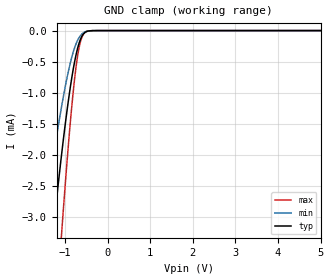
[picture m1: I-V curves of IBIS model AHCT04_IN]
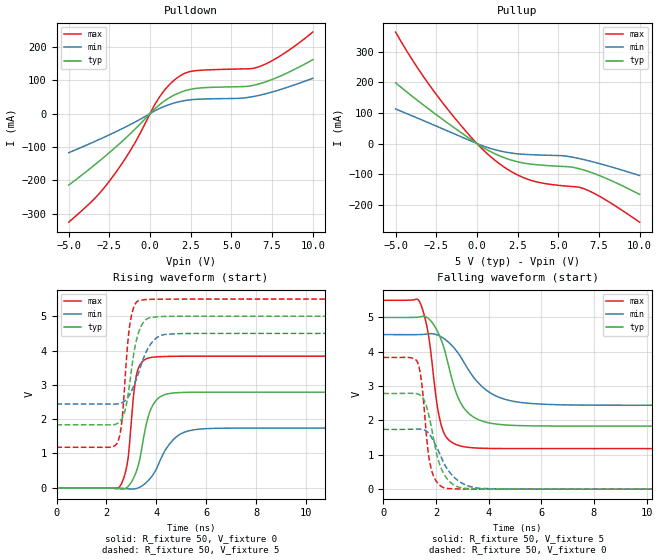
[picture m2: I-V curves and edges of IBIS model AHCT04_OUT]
| TEXAS INSTRUMENTS INCORPORATED
| Standard Linear and Logic Group
| IBIS Model of SN74AHCT1G04
| SINGLE INVERTER GATE
| This file contains package information for the following:
|  SOT 5-pin (DBV) package as [Component] AHCT04_DBV
|  SOT 5-pin (DCK) package as [Component] AHCT04_DCK
| This device can be powered at the following Vccs:
|  5 volt Vcc
| This file provides unique models under the [Model Selector] for each Vcc.
| For operation at a specific Vcc, select the appropriate model after each
| [Model Selector] keyword.
[IBIS Ver]   3.2
[Comment char]  |_char
[File Name]   sn74ahct1g04.ibs
[File Rev]   1.1 | j_die
[Date]   October 25, 2007
[Source]   Data created from TI-SPICE simulations at TI-SLL.
[Notes]   The following is an IBIS list for the SN74AHCT1G04.
   Please contact sllibis@ti.com with questions and
   comments concerning SLL IBIS models.
   - FILE REV HISTORY
   - 1.1 Release IBIS file on 11/9/07
   - Power clamp data deleted as there is no power-clamp diode.
[Disclaimer] Property of Texas Instruments Incorporated.  Unauthorized
   reproduction and/or distribution is strictly prohibited.
   This product is protected under copyright law.
   Created  2007, (C) Copyright  2007, Texas Instruments
   Incorporated, All Rights Reserved
   UNLESS THERE IS A SIGNED, WRITTEN AGREEMENT TO THE
   CONTRARY, TEXAS INSTRUMENTS (TI) IS PROVIDING THE IBIS
   MODELS  AND WITHOUT ANY WARRANTY, EXPRESSED OR
   IMPLIED.  TI assumes no liability for:
   1) the accuracy of the IBIS models provided to your
   company;
   2) the proper functioning of these IBIS Models in your
   design or for any resulting applications; or
   3) infringement of patents, copyrights or intellectual
   property rights resulting from your use of these IBIS
   models.
   TI provides IBIS Models as a service to our customers.
   You and your company shall not distribute, sell or give
   these models to anyone else without prior written
   permission from TI.
   TI reserves the right to make changes to our products or
   to discontinue any semiconductor product or service
   without notice, and advises our customers to obtain the
   latest version of relevant information to verify, before
   placing orders, that the information being relied on is
   current.
   Please be aware that your receipt and use of the IBIS
   information provided shall serve as acceptance of these
   terms and conditions.  If you do not accept these terms,
   you should return or destroy the IBIS models and any
   other accompanying information immediately.
| Component SN74AHCT1G04_DBV 5-PIN SOT
[Component]   SN74AHCT1G04_DBV
[Manufacturer]   Texas Instruments, Inc.
[Package]
|   typ   min   max
R_pkg   2.500e-02   2.100e-02   2.900e-02
L_pkg   1.529e-09   1.312e-09   1.906e-09
C_pkg   1.560e-13   1.100e-13   2.400e-13
[Pin]   signal_name   model_name   R_pin   L_pin   C_pin
1   NC   NC   2.100e-02   1.511e-09   1.440e-13
2   A   AHCT04_IN   2.300e-02   1.312e-09   1.380e-13
3   GND   GND   2.900e-02   1.906e-09   2.400e-13
4   Y   AHCT04_OUT   2.600e-02   1.541e-09   1.500e-13
5   VCC   POWER   2.500e-02   1.374e-09   1.100e-13
| Component SN74AHCT1G04_DCK 5-PIN SOT
[Component]   SN74AHCT1G04_DCK
[Manufacturer]   Texas Instruments, Inc.
[Package]
|   typ   min   max
R_pkg   2.000e-02   1.700e-02   2.500e-02
L_pkg   9.980e-10   8.810e-10   1.069e-09
C_pkg   1.460e-13   1.180e-13   2.050e-13
[Pin]   signal_name   model_name   R_pin   L_pin   C_pin
1   NC   NC   1.900e-02   1.069e-09   1.620e-13
2   A   AHCT04_IN   1.800e-02   8.810e-10   1.210e-13
3   GND   GND   1.700e-02   1.031e-09   2.050e-13
4   Y   AHCT04_OUT   2.000e-02   9.600e-10   1.240e-13
5   VCC   POWER   2.500e-02   1.049e-09   1.180e-13
| Models and submodels in the file (2): AHCT04_IN (Input), AHCT04_OUT (Output)
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[Model]   AHCT04_IN
Model_type  Input
Vinl=0.8
Vinh=2.0
| variable   typ   min   max
C_comp   1.07pF   0.88pF   1.17pF
[Temperature Range]   40   100   -40
| Ambient temperature   25   85   -40
[Voltage range]   5   4.5   5.5
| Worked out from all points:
|   GND clamp passes 1 mA (typ) near -0.89 V on its own axis
[GND Clamp]
| AHCT04_IN
|   Voltage   I(typ)   I(min)   I(max)
-5V       -39.05mA   -25.88mA   -50.64mA
-1.54V    -5.118mA   -3.294mA   -8.041mA
-1.49V    -4.743mA   -3.046mA   -7.491mA
-1.28V    -3.254mA   -2.059mA   -5.253mA
-1.08V    -1.989mA   -1.219mA   -3.261mA
-900mV    -1.024mA   -591uA     -1.667mA
-775mV    -501.2uA   -275.4uA   -773.8uA
-720mV    -326.3uA   -178.4uA   -476uA
-660mV    -181.4uA   -102.3uA   -240.9uA
-610mV    -98.63uA   -59.63uA   -118uA
-540mV    -34.66uA   -23.86uA   -34.5uA
5V        17.64nA    1.142nA    163.4nA
[Model]   AHCT04_OUT
Model_type  Output
Vref =   0
Rref =   1000
Cref =   50p
Vmeas =   1.5
| variable   typ   min   max
C_comp   3.84pF   2.05pF   6.98pF
| C_pullup   3.33pF   2.05pF   4.35pF
| C_pulldown   4.35pF   2.74pF   6.98pF
[Temperature Range]   40   100   -40
| Ambient temperature   25   85   -40
[Voltage range]   5   4.5   5.5
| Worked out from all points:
|   slope of the pulldown table from 0 to 0.75 V, typ, clamps not added: 22.7 ohm
|   slope of the pullup table from 0 to 0.75 V, typ, clamps not added: 31.3 ohm
|   rising waveform, R_fixture 50, V_fixture 0: 20-80 % time 509ps typ, 836ps min, 304ps max; typ from 0 V to 2.79 V
|   falling waveform, R_fixture 50, V_fixture 5: 20-80 % time 783ps typ, 1.25ns min, 462ps max; typ from 5 V to 1.84 V
|   rising waveform, R_fixture 50, V_fixture 5: 20-80 % time 414ps typ, 660ps min, 281ps max; typ from 1.84 V to 5 V
|   falling waveform, R_fixture 50, V_fixture 0: 20-80 % time 522ps typ, 776ps min, 309ps max; typ from 2.79 V to 0 V
[Pulldown]
| AHCT04_OUT
|   Voltage   I(typ)   I(min)   I(max)
-5V       -214.3mA   -117.4mA   -325.8mA
-3.425V   -154.6mA   -84.24mA   -255.7mA
-2.375V   -111.7mA   -60.8mA    -194.5mA
-1.035V   -51.93mA   -28.28mA   -96.41mA
515mV     23.92mA    13.69mA    44.79mA
1.035V    42.89mA    24.61mA    78.63mA
1.59V     58.05mA    33.27mA    104.4mA
2.66V     74.47mA    42.18mA    127.9mA
5.55V     80.78mA    45.98mA    134mA
6.665V    88.69mA    54.35mA    140.1mA
8.135V    115.3mA    74.05mA    177.2mA
10V       161.8mA    105.9mA    244.5mA
[Pullup]
| AHCT04_OUT
|   Voltage   I(typ)   I(min)   I(max)
-5V       198.5mA    112.9mA    364.5mA
-3.58V    138mA      81.55mA    241.8mA
-2V       74.74mA    45.71mA    125.7mA
-170mV    6.077mA    3.809mA    9.646mA
1.225V    -36.41mA   -21.83mA   -59.68mA
2.27V     -56.59mA   -32.28mA   -96.46mA
3.315V    -67.32mA   -36.47mA   -120.2mA
5.32V     -75.07mA   -40.25mA   -138.4mA
6.22V     -81.58mA   -48.34mA   -142.5mA
6.76V     -89.85mA   -54.93mA   -151.7mA
8.04V     -116.3mA   -73.18mA   -188.4mA
10V       -166.4mA   -104.7mA   -257.3mA
[Ramp]
| AHCT04_OUT
| variable   typ   min   max
dV/dt_r   1.70/5.27E-10   1.07/8.58E-10   2.32/3.15E-10
dV/dt_f   1.92/7.95E-10   1.25/1.27E-09   2.61/4.73E-10
R_load = 50
[Rising Waveform]
| AHCT04_OUT
R_fixture =   50
C_fixture =   0
L_fixture =   0
V_fixture =   0
V_fixture_min = 0
V_fixture_max = 0
|   Time   V(typ)   V(min)   V(max)
0s        151.2pV    237.8pV    69.57pV
2.54ns    -30.49mV   -10.33mV   43.03mV
2.865ns   36.16mV    -29.86mV   840.8mV
3.08ns    267.7mV    -34.84mV   2.638V
3.22ns    517.7mV    -16.51mV   3.337V
3.74ns    2.217V     262.4mV    3.791V
4.11ns    2.627V     721.9mV    3.82V
4.7ns     2.763V     1.416V     3.832V
5.72ns    2.785V     1.709V     3.836V
24.99ns   2.787V     1.74V      3.836V
[Falling Waveform]
| AHCT04_OUT
R_fixture =   50
C_fixture =   0
L_fixture =   0
V_fixture =   5
V_fixture_min = 4.5
V_fixture_max = 5.5
|   Time   V(typ)   V(min)   V(max)
0s        5V         4.5V       5.5V
1.375ns   5.016V     4.502V     5.458V
1.695ns   4.98V      4.522V     4.567V
2.015ns   4.654V     4.499V     2.586V
2.21ns    4.32V      4.43V      1.831V
2.465ns   3.629V     4.284V     1.445V
2.985ns   2.449V     3.793V     1.248V
4.04ns    1.926V     2.813V     1.186V
5.61ns    1.844V     2.494V     1.181V
24.99ns   1.837V     2.443V     1.181V
[Rising Waveform]
| AHCT04_OUT
R_fixture =   50
C_fixture =   0
L_fixture =   0
V_fixture =   5
V_fixture_min = 4.5
V_fixture_max = 5.5
|   Time   V(typ)   V(min)   V(max)
0s        1.837V     2.443V     1.181V
2.425ns   1.87V      2.442V     1.296V
2.625ns   2.02V      2.481V     1.973V
2.835ns   2.563V     2.609V     4.049V
2.94ns    3.079V     2.727V     4.758V
3.125ns   4.031V     3.024V     5.313V
3.32ns    4.589V     3.42V      5.459V
3.795ns   4.962V     4.21V      5.493V
4.4ns     4.995V     4.472V     5.498V
24.99ns   5V         4.5V       5.5V
[Falling Waveform]
| AHCT04_OUT
R_fixture =   50
C_fixture =   0
L_fixture =   0
V_fixture =   0
V_fixture_min = 0
V_fixture_max = 0
|   Time   V(typ)   V(min)   V(max)
0s        2.787V     1.74V      3.836V
1.29ns    2.776V     1.749V     3.706V
1.445ns   2.71V      1.743V     3.15V
1.675ns   2.313V     1.663V     1.26V
1.8ns     1.895V     1.542V     645.9mV
2.07ns    886mV      1.147V     170.5mV
2.37ns    356.2mV    658mV      26.71mV
2.96ns    36.75mV    187.8mV    4.835mV
3.78ns    6.232mV    20.45mV    552.8uV
24.99ns   -9.814nV   -17.55nV   -667.9pV
